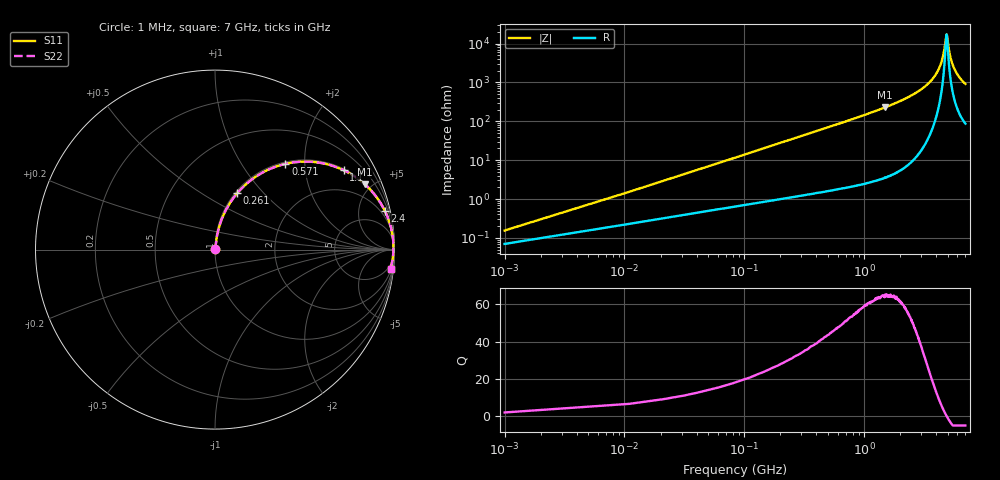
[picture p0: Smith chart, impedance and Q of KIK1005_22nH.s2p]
!version-3
!date-01.2023
!Series
# MHz S RI R 50
!Freq ReS11 ImS11 ReS21 ImS21 ReS12 ImS12 ReS22 ImS22
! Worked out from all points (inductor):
!   701 points, 1 MHz to 7 GHz, reference 50 ohm
!   read as one part in series: L = 22 nH near 31 MHz
!   highest Q = 64.8 at 1.49 GHz (marker M1), where L = 24.3 nH
!   self-resonance near 4.88 GHz
!   S11 on the Smith chart (normalised r, x): 1 MHz: 1.00, +0.00; 261 MHz: 1.02, +0.72; 571 MHz: 1.03, +1.60; 1.1 GHz: 1.05, +3.21; 2.4 GHz: 1.16, +8.75; 7 GHz: 3, -18
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1  0.000701 0.00138  0.9993 -0.00138  0.9993 -0.00138  0.000701 0.00138
41  0.00762 0.056  0.9924 -0.056  0.9924 -0.056  0.00762 0.056
71  0.0152 0.0961  0.9848 -0.0961  0.9848 -0.0961  0.0152 0.0961
141  0.044 0.1849  0.956 -0.1849  0.956 -0.1849  0.044 0.1849
261  0.1234 0.3136  0.8766 -0.3136  0.8766 -0.3136  0.1234 0.3136
571  0.3927 0.4777  0.6073 -0.4777  0.6073 -0.4777  0.3927 0.4777
1100  0.7168 0.4424  0.2832 -0.4424  0.2832 -0.4424  0.7168 0.4424
1170  0.7434 0.4287  0.2566 -0.4287  0.2566 -0.4287  0.7434 0.4287
1490  0.8341 0.3644  0.1659 -0.3644  0.1659 -0.3644  0.8341 0.3644
2340  0.9428 0.2233  0.0572 -0.2233  0.0572 -0.2233  0.9428 0.2233
2400  0.9468 0.2153  0.0532 -0.2153  0.0532 -0.2153  0.9468 0.2153
3510  0.9861 0.0977  0.0139 -0.0977  0.0139 -0.0977  0.9861 0.0977
4250  0.9934 0.0407  0.00657 -0.0407  0.00657 -0.0407  0.9934 0.0407
4490  0.9942 0.0245  0.00582 -0.0245  0.00582 -0.0245  0.9942 0.0245
4670  0.9944 0.013  0.00564 -0.013  0.00564 -0.013  0.9944 0.013
4830  0.9943 0.00314  0.00572 -0.00314  0.00572 -0.00314  0.9943 0.00314
4890  0.9942 -0.000471  0.00581 0.000471  0.00581 0.000471  0.9942 -0.000471
5110  0.9936 -0.0133  0.00635 0.0133  0.00635 0.0133  0.9936 -0.0133
5270  0.993 -0.0223  0.00696 0.0223  0.00696 0.0223  0.993 -0.0223
5510  0.9918 -0.0353  0.00816 0.0353  0.00816 0.0353  0.9918 -0.0353
5840  0.9897 -0.0523  0.0103 0.0523  0.0103 0.0523  0.9897 -0.0523
7000  0.9784 -0.1053  0.0216 0.1053  0.0216 0.1053  0.9784 -0.1053
